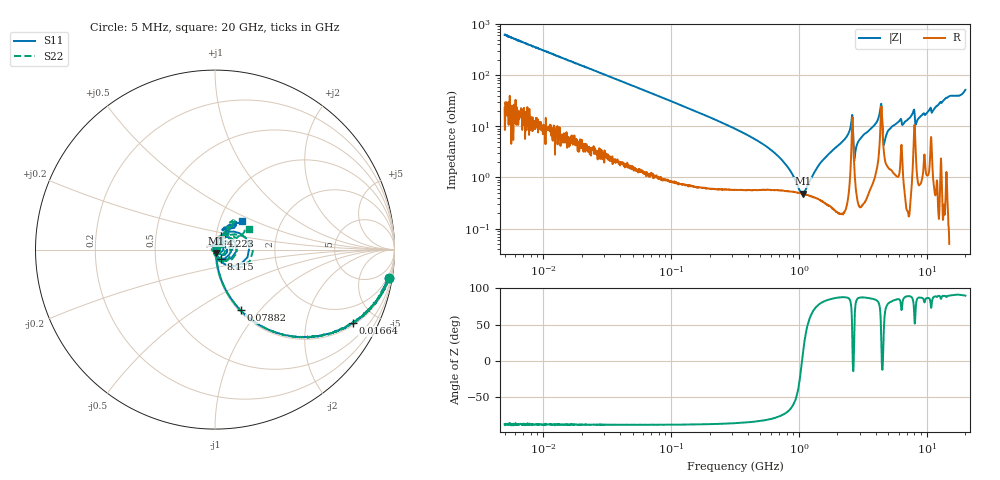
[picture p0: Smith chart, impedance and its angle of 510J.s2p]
!Keysight Technologies,P5008B,MY61100088,A.16.20.02
!Date: Wednesday, November 08, 2023 15:16:56
!Correction: S11(C  2-Port  )
!S21(C  2-Port  )
!S12(C  2-Port  )
!S22(C  2-Port  )
!S2P File: Measurements: S11, S21, S12, S22:Log Frequency Sweep
# Hz S  dB  R 50
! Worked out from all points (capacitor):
!   1601 points, 5 MHz to 20 GHz, reference 50 ohm
!   read as one part in series: C = 51.8 pF near 5.212 MHz
!   lowest |Z| = 481 mohm at 1.069 GHz (marker M1)
!   series resonance near 1.057 GHz, so ESL is about 440 pH
!   S11 on the Smith chart (normalised r, x): 5 MHz: 1, -12; 16.64 MHz: 1.09, -3.72; 78.82 MHz: 1.02, -0.79; 4.223 GHz: 1.06, +0.17; 8.115 GHz: 1.07, -0.11; 20 GHz: 1.28, +0.43
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5000000  -0.16 -9.1  -15.97 78.7  -15.97 78.7  -0.16 -9.1
1.664442e7  -1.19 -27.9  -6.59 60.6  -6.59 60.6  -1.19 -28.0
1.995555e7  -1.60 -32.3  -5.44 56.3  -5.44 56.3  -1.60 -32.3
7.882336e7  -8.73 -67.1  -0.71 21.3  -0.71 21.3  -8.74 -67.2
7.964482e7  -8.81 -67.4  -0.69 21.1  -0.70 21.1  -8.81 -67.5
3.162278e8  -20.50 -81.3  -0.09 4.8  -0.09 4.8  -20.68 -82.2
1.069184e9  -34.28 -79.2  -0.06 -1.0  -0.06 -1.0  -37.27 -85.6
1.2621e9  -36.63 -81.6  -0.06 -1.8  -0.06 -1.7  -40.74 -92.5
1.56909e9  -44.54 -100.1  -0.06 -2.8  -0.07 -2.8  -54.96 -142.0
1.758637e9  -52.46 -171.2  -0.07 -3.5  -0.07 -3.5  -48.13 123.4
2.594315e9  -19.56 40.1  -0.82 -9.5  -0.82 -9.5  -19.46 34.5
2.953282e9  -39.21 143.3  -0.09 -5.9  -0.09 -5.9  -54.23 85.2
4.22322e9  -21.39 66.2  -0.31 -12.9  -0.32 -12.9  -20.84 51.1
4.49427e9  -18.70 -50.2  -0.82 -3.6  -0.83 -3.6  -17.79 -48.5
5.037181e9  -45.45 -7.5  -0.12 -9.6  -0.13 -9.6  -31.59 -7.3
6.197821e9  -29.99 42.7  -0.21 -14.1  -0.21 -14.1  -32.69 52.5
7.092062e9  -40.40 34.4  -0.12 -15.4  -0.12 -15.4  -32.24 145.2
8.115326e9  -24.08 -56.7  -0.55 -14.4  -0.56 -14.4  -22.95 -66.7
8.955306e9  -45.52 -67.8  -0.08 -18.9  -0.08 -18.9  -37.73 -61.9
1.136684e10  -32.75 25.1  -0.06 -24.5  -0.07 -24.4  -33.22 70.1
1.405861e10  -15.36 52.3  -0.11 -32.6  -0.11 -32.6  -15.88 54.5
2e10  -13.11 46.2  -0.28 -52.1  -0.28 -52.1  -13.17 30.7
